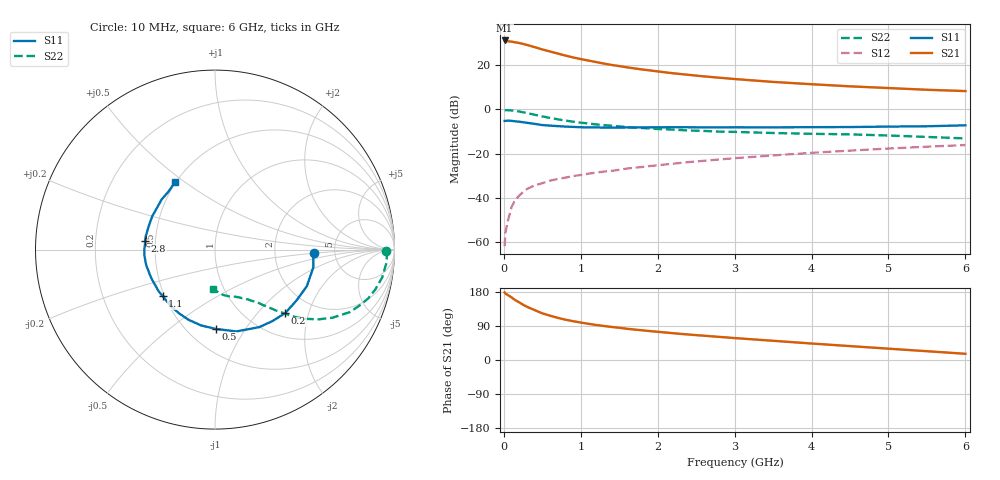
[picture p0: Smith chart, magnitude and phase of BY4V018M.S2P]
! SIEMENS Small Signal Semiconductors
! BFY420
! Si NPN RF SIEGET Grounded Emitter Transistor in MICRO-X
! VCE = 4 V  IC = 18 mA
! Common Emitter S-Parameters:  October  1996
# GHz  S  MA  R  50
!  f  S11  S21  S12  S22
! GHz  MAG  ANG  MAG  ANG  MAG  ANG  MAG  ANG
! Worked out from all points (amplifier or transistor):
!   36 points, 10 MHz to 6 GHz, reference 50 ohm
!   highest |S21| = 31.2 dB at 10 MHz (marker M1)
!   |S21| within 3 dB of that: start of sweep to 399 MHz
!   unconditionally stable (mu >= 1): start of sweep to 16.64 MHz; 2.074 GHz to end of sweep
!   at 250 MHz: K = 0.32, MSG = 33.5 dB, |S12| = -37.4 dB
!   at 1.4 GHz: K = 0.89, MSG = 24.0 dB, |S12| = -27.9 dB
!   at 6 GHz: K = 1.06, MAG = 10.7 dB, |S12| = -16.1 dB
!   S11 on the Smith chart (normalised r, x): 10 MHz: 3.42, -0.20; 200 MHz: 1.46, -1.43; 500 MHz: 0.68, -0.74; 1.1 GHz: 0.49, -0.30; 2.8 GHz: 0.44, +0.05; 6 GHz: 0.49, +0.46
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0.01  0.5492 -2.1  36.38 178.2  0.0008 45.4  0.9543 -0.4
0.02  0.5494 -4.2  35.85 175.5  0.0016 44.4  0.9592 -1.4
0.1  0.5509 -21.7  34.2 165.3  0.0061 74.1  0.9446 -9.4
0.15  0.5356 -31.7  32.97 157.7  0.0091 71.5  0.9214 -13.8
0.2  0.5276 -42.1  31.86 152.1  0.0112 71.7  0.895 -17.8
0.25  0.5106 -51.4  30.39 145.8  0.0135 66.9  0.8591 -21.6
0.3  0.4974 -60.3  28.79 140.5  0.0157 66.1  0.8275 -24.9
0.4  0.4712 -75.4  25.72 131.7  0.019 62.6  0.7566 -30.1
0.5  0.4419 -89.5  22.76 123.1  0.0213 60.5  0.695 -34.0
0.6  0.4294 -100.5  20.45 117.0  0.0243 59.6  0.6414 -37.0
0.7  0.418 -110.4  18.41 111.3  0.0266 59.0  0.5969 -39.4
0.8  0.4081 -119.0  16.56 106.4  0.0285 57.4  0.5579 -41.2
0.9  0.4015 -125.5  15.01 102.4  0.031 57.0  0.527 -42.4
1.1  0.3904 -138.5  12.76 95.5  0.035 57.8  0.4777 -45.1
1.3  0.3876 -147.6  10.92 89.8  0.039 57.7  0.4401 -47.0
1.6  0.3892 -158.9  8.956 82.4  0.0458 57.9  0.398 -49.8
2.2  0.3944 -175.1  6.576 70.7  0.059 57.0  0.3479 -54.8
2.8  0.392 172.6  5.214 61.0  0.0735 54.6  0.3138 -59.5
3.5  0.3917 160.1  4.191 50.7  0.0907 50.7  0.292 -64.9
4.5  0.3982 144.3  3.326 36.7  0.1166 43.5  0.2719 -73.4
5.5  0.4148 128.4  2.781 23.2  0.1431 35.1  0.2379 -85.5
6  0.4358 120.9  2.6 16.4  0.1558 30.5  0.2203 -93.3
